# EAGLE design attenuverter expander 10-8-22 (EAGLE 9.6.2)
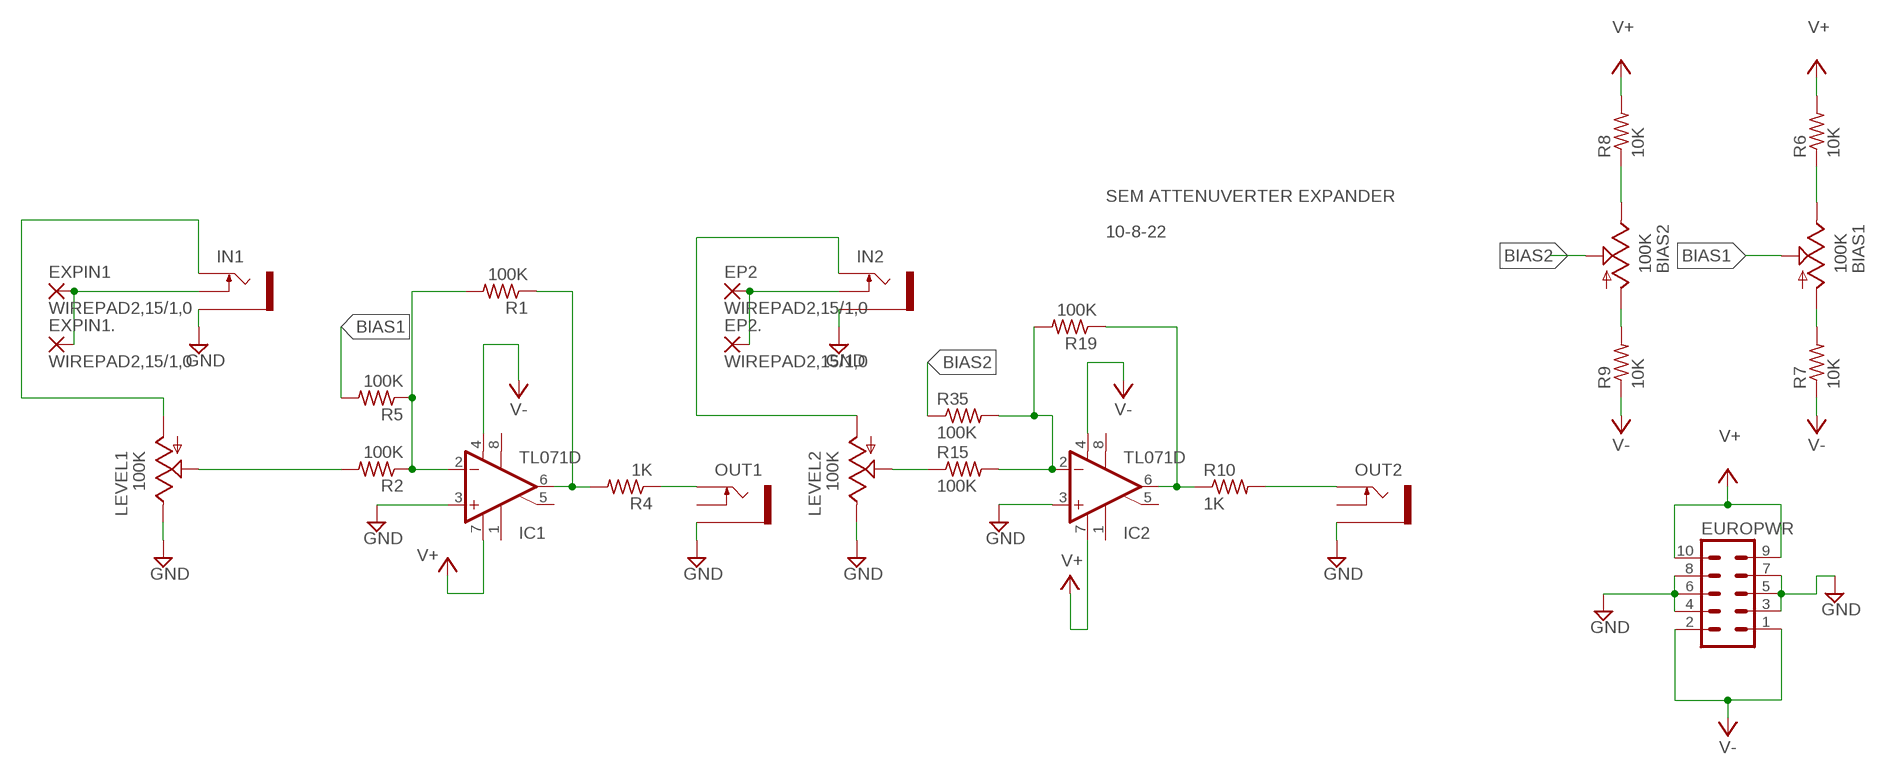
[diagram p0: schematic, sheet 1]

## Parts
BIAS1  100K  9MM_SNAP-IN_POT_  [9MM_SNAP-IN_POT]
BIAS2  100K  9MM_SNAP-IN_POT_  [9MM_SNAP-IN_POT]
EP2  WIREPAD2,15/1,0  [2,15/1,0]
EP2.  WIREPAD2,15/1,0  [2,15/1,0]
EUROPWR  EURO_POWER_HEADERREGULAR  [EURO_POWER_HEADER]
EXPIN1  WIREPAD2,15/1,0  [2,15/1,0]
EXPIN1.  WIREPAD2,15/1,0  [2,15/1,0]
IC1  TL071D  [SO08]
IC2  TL071D  [SO08]
IN1  THONKICONNNEW  [WQP-PJ301M-12_JACK]
IN2  THONKICONNNEW  [WQP-PJ301M-12_JACK]
LEVEL1  100K  9MM_SNAP-IN_POT_  [9MM_SNAP-IN_POT]
LEVEL2  100K  9MM_SNAP-IN_POT_  [9MM_SNAP-IN_POT]
OUT1  THONKICONNNEW  [WQP-PJ301M-12_JACK]
OUT2  THONKICONNNEW  [WQP-PJ301M-12_JACK]
R1  100K  R-US_0204/7  [0204/7]
R2  100K  R-US_0204/7  [0204/7]
R4  1K  R-US_0204/7  [0204/7]
R5  100K  R-US_0204/7  [0204/7]
R6  10K  R-US_0204/7  [0204/7]
R7  10K  R-US_0204/7  [0204/7]
R8  10K  R-US_0204/7  [0204/7]
R9  10K  R-US_0204/7  [0204/7]
R10  1K  R-US_0204/2V  [0204V]
R15  100K  R-US_0204/7  [0204/7]
R19  100K  R-US_0204/7  [0204/7]
R35  100K  R-US_0204/2V  [0204V]

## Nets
BIAS1: BIAS1.2(S) R5.2
BIAS2: BIAS2.2(S) R35.1
GND: EUROPWR.3 EUROPWR.4 EUROPWR.5 EUROPWR.6 EUROPWR.7 EUROPWR.8 IC1.3(+IN) IC2.3(+IN) IN1.P$3_SLEEVE(SLEEVE) IN2.P$3_SLEEVE(SLEEVE) LEVEL1.3(E) LEVEL2.3(E) OUT1.P$3_SLEEVE(SLEEVE) OUT2.P$3_SLEEVE(SLEEVE)
N$1: BIAS2.3(E) R8.1
N$2: BIAS2.1(A) R9.2
N$3: BIAS1.1(A) R7.2
N$4: BIAS1.3(E) R6.1
N$5: IC1.2(-IN) R1.2 R2.1 R5.1
N$6: IC1.6(OUT) R1.1 R4.2
N$7: IC2.2(-IN) R15.2 R19.2 R35.2
N$8: LEVEL1.2(S) R2.2
N$9: IC2.6(OUT) R10.1 R19.1
N$10: LEVEL2.2(S) R15.1
N$11: EXPIN1.1(P) EXPIN1..1(P) IN1.P$2_SWITCH(SWITCH)
N$12: EP2.1(P) EP2..1(P) IN2.P$2_SWITCH(SWITCH)
N$13: IN2.P$1_TIP(TIP) LEVEL2.1(A)
N$14: IN1.P$1_TIP(TIP) LEVEL1.1(A)
N$15: OUT2.P$1_TIP(TIP) R10.2
N$16: OUT1.P$1_TIP(TIP) R4.1
V+: EUROPWR.9 EUROPWR.10 IC1.7(V+) IC2.7(V+) R6.2 R8.2
V-: EUROPWR.1 EUROPWR.2 IC1.4(V-) IC2.4(V-) R7.1 R9.1
Unconnected: IC1.1(ON1) IC1.5(ON2) IC1.8(OPT) IC2.1(ON1) IC2.5(ON2) IC2.8(OPT) OUT1.P$2_SWITCH(SWITCH) OUT2.P$2_SWITCH(SWITCH)

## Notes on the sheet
- SEM ATTENUVERTER EXPANDER
- 10-8-22

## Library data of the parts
BIAS1 BIAS2 LEVEL1 LEVEL2 = MusicThingModular:9MM_SNAP-IN_POT: 9mm vertical snap-in pot, Alpha / Panasonic style
EP2 EP2. EXPIN1 EXPIN1. = wirepad:WIREPAD: Wire PAD connect wire on PCB
EUROPWR = MusicThingModular:EURO_POWER_HEADER: Power Header 10 pin power header for Eurorack Power Supplies Variants with fatter pads for easier soldering, and the LOCK variant which has 5mil offset pins to hold the component in place before soldering
IC1 IC2 = linear:TL071: OP AMP
IN1 IN2 OUT1 OUT2 = MusicThingModular-CL:THONKICONN: 3.5mm socket for Eurorack modular synths
R1 R2 R4 R5 = rcl:R-US_: RESISTOR, American symbol
R6-R10 R15 R19 R35 = adafruit:R-US_: RESISTOR, American symbol

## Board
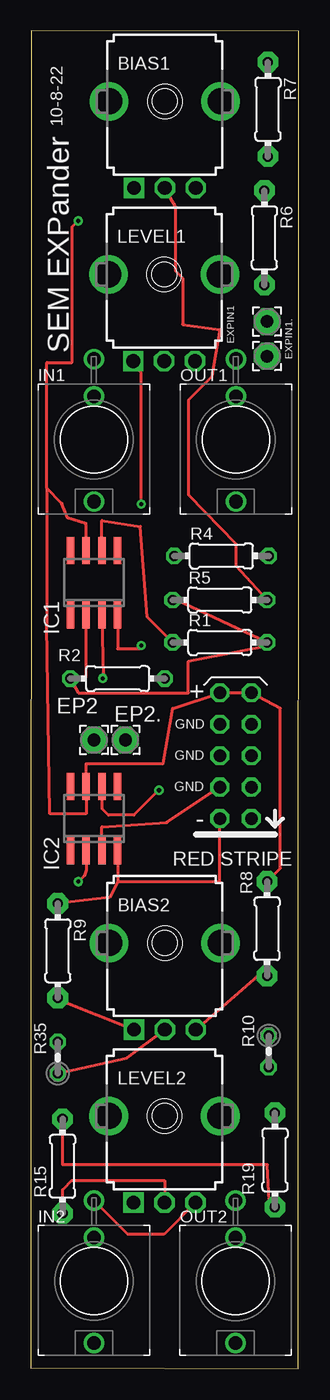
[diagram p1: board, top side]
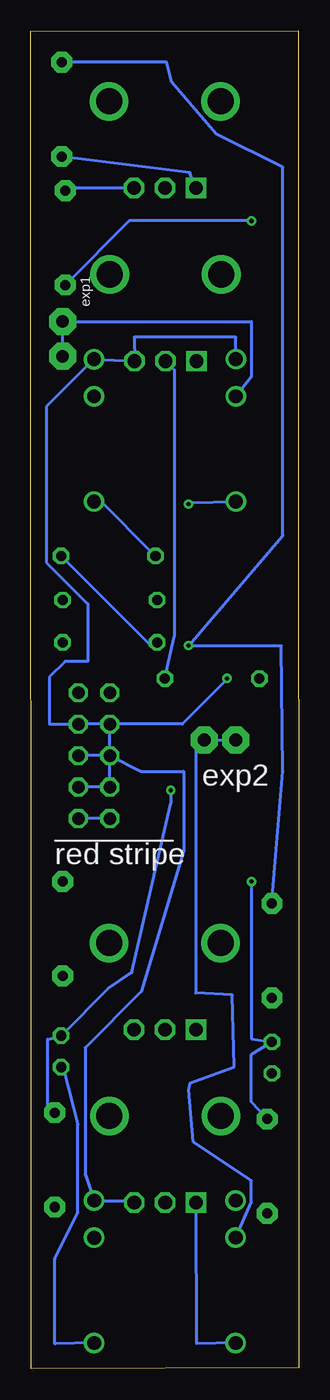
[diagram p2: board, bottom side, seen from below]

Size 21.61 x 108 mm. Coordinates in mm from the lower left corner, seen from the top.
Outline: 0,0.06 21.59,0 21.61,108 0.02,108 0,0.06
Copper layers (1*16): Top 0.035mm / dielectric 1.5mm / Bottom 0.035mm
Design rules "default": minimum track width 6mil, minimum drill 0.35mm, track to track 6mil, track to pad 6mil, pad to pad 6mil, via to via 6mil, smd to smd 6mil, copper to edge 40mil, drill to drill 6mil, minimum pad ring 10mil, minimum via ring 8mil, stop-mask expansion 4mil, vias tented up to drill 0mil, thermal gap 10mil

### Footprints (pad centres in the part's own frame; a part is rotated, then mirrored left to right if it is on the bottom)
9MM_SNAP-IN_POT = drill 1.1 square: 1 -2.5,-7 | drill 1.1 octagon: 2 0,-7; 3 2.5,-7 | drill 2.1 pad 2.794: CHASSIS1 -4.5,0; CHASSIS2 4.5,0
2,15/1,0 = drill 1.016 pad 2.159 octagon: 1 0,0
EURO_POWER_HEADER = drill 1.016 octagon: 1 -5.08,-1.27; 2 -5.08,1.27; 3 -2.54,-1.27; 4 -2.54,1.27; 5 0,-1.27; 6 0,1.27; 7 2.54,-1.27; 8 2.54,1.27; 9 5.08,-1.27; 10 5.08,1.27
SO08 = smd 0.6 x 2.2: 1 -1.905,-2.6; 2 -0.635,-2.6; 3 0.635,-2.6; 4 1.905,-2.6; 5 1.905,2.6; 6 0.635,2.6; 7 -0.635,2.6; 8 -1.905,2.6
WQP-PJ301M-12_JACK = drill 1.1: P$1_TIP 0,5; P$2_SWITCH 0,-3.5; P$3_SLEEVE 0,-6.5
0204/7 = drill 0.813 octagon: 1 -3.81,0; 2 3.81,0
0204/7' = drill 0.813 pad 1.676 octagon: 1 -3.81,0; 2 3.81,0
0204V = drill 0.813 octagon: 1 -1.27,0; 2 1.27,0

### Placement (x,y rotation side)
BIAS1  10.8,102.32 0 top
BIAS2  10.8,34.36 0 top
EP2  5.09,50.76 0 top
EP2.  7.63,50.76 0 top
EUROPWR  16.52,49.49 90 top
EXPIN1  19.06,81.74 0 top
EXPIN1.  19.06,84.54 0 top
IC1  5.09,63.46 0 top
IC2  5.09,44.41 0 top
IN1  5.08,75 180 top
IN2  5.09,7.07 180 top
LEVEL1  10.75,88.35 0 top
LEVEL2  10.78,20.39 0 top
OUT1  16.54,75 180 top
OUT2  16.51,7.06 180 top
R1  15.25,58.63 0 top
R2  6.99,55.71 0 top
R4  15.37,65.61 0 top
R5  15.25,62.06 0 top
R6  10K  [0204/7']  18.84,91.3 270 top
R7  10K  [0204/7']  19.13,101.68 270 top
R8  10K  [0204/7']  19.06,35.52 90 top
R9  10K  [0204/7']  2.17,33.74 270 top
R10  19.18,25.61 270 top
R15  100K  [0204/7']  2.55,16.34 90 top
R19  100K  [0204/7']  19.69,16.85 270 top
R35  2.17,25.1 90 top

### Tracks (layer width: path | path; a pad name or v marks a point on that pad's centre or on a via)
BIAS1
  Top 0.254: R5.2 16.52,64.82 16.52,66.63 12.71,70.57 12.71,78.19 14.61,80.09 15.25,83.9 12.24,84.3 12.24,88.06 11.69,88.6 11.69,93.77 BIAS1.2
BIAS2
  Top 0.254: R35.1 7.77,25.1 BIAS2.2
GND  (via drill 0.35)
  Top 0.254: IC1.3 5.84,55.69 v5.79,55.72 | IC2.3 5.72,43.74 10.97,44.09 EUROPWR.4 | LEVEL2.3 10.74,10.85 7.81,10.85 IN2.P$3_SLEEVE
  Bottom 0.254: IN1.P$3_SLEEVE 5.08,83.27 13.29,83.27 13.25,81.36 | 13.25,81.36 LEVEL1.3 | v5.79,55.72 5.79,55.63 9.39,52.03 EUROPWR.8 | EUROPWR.8 EUROPWR.7 20.12,52.03 20.12,55.84 18.85,57.11 17.02,57.11 17.02,61.75 20.38,65.1 20.38,77.66 OUT1.P$3_SLEEVE 13.25,81.36 | EUROPWR.6 EUROPWR.8 | EUROPWR.6 EUROPWR.5 | EUROPWR.6 EUROPWR.4 EUROPWR.3 | LEVEL2.3 13.45,13.56 OUT2.P$3_SLEEVE 17.24,15.67 17.24,25.9 12.71,30.44 9.28,41.85 9.28,48.22 12.71,48.22 EUROPWR.6
N$1
  Top 0.254: R8.1 18.29,31.71 BIAS2.3
N$2
  Top 0.254: BIAS2.1 2.4,29.7 R9.2
N$3
  Bottom 0.254: BIAS1.1 8.79,96.57 R7.2
N$4
  Bottom 0.254: R6.1 18.16,95.32 BIAS1.3
N$5
  Top 0.254: IC1.2 4.45,55.84 R2.1 3.82,54.57 12.71,54.57 12.71,57.11 18.7,58.28 R1.2 11.73,62.06 R5.1
N$6
  Top 0.254: IC1.6 5.72,68.49 8.82,68 9.4,60.67 R1.1
  Bottom 0.254: R4.2 11.84,58.27 R1.1
N$7  (via drill 0.35)
  Top 0.254: IC2.2 4.46,40.24 4.29,39.8 v3.82,39.33 | R19.2 19.24,13.49 19.07,16.47 2.55,16.47 R15.2
  Bottom 0.254: R15.2 3.82,21.55 3.82,25.36 R35.2 3.82,26.63 v3.82,39.33
N$8
  Bottom 0.254: R2.2 10.03,59.12 10.03,80.62 LEVEL1.2
N$9  (via drill 0.35)
  Top 0.254: IC2.6 5.72,45.22 6.26,44.68 8.3,44.68 v10.33,46.7
  Bottom 0.254: R19.1 20.27,21.23 20.27,26.59 R10.1 15.38,30.68 13.48,31.98 10.33,45.63 v10.33,46.7
N$10
  Top 0.254: R15.1 2.55,14.43 3.31,15.2 10.78,15.2 LEVEL2.2
N$11
  Bottom 0.254: IN1.P$2_SWITCH 3.82,80.08 3.82,84.54 EXPIN1..1 EXPIN1.1
N$12
  Bottom 0.254: EP2.1 EP2..1 8.32,50.06 8.32,30.33 5.35,30.17 5.22,24.36 8.75,23.06 8.89,22.52 8.5,18.31 3.82,15.2 3.82,13.42 IN2.P$2_SWITCH
N$13
  Bottom 0.254: IN2.P$1_TIP 8.24,2 LEVEL2.1
N$14  (via drill 0.35)
  Top 0.254: v8.9,69.81 8.9,80.36 LEVEL1.1
  Bottom 0.254: IN1.P$1_TIP 8.78,69.93 v8.9,69.81
N$15
  Bottom 0.254: OUT2.P$1_TIP 19.69,1.99 19.69,8.85 17.82,12.59 17.82,19.71 18.98,24.14 R10.2
N$16
  Bottom 0.254: OUT1.P$1_TIP 16.2,70.25 R4.1
V+  (via drill 0.35)
  Top 0.254: 1.28,71.08 2.5,69.85 2.97,68.69 4.44,68.25 4.45,68.03 IC1.7 | 1.28,71.08 1.28,81.24 3.31,81.24 3.31,92.16 v3.82,92.67 | 1.28,71.08 1.28,60.03 1.53,44.79 4.45,44.79 IC2.7 4.45,48.85 10.67,48.85 11.44,53.3 EUROPWR.10 EUROPWR.9 20.12,53.3 20.12,40.39 R8.2
  Bottom 0.254: v3.82,92.67 13.67,92.67 R6.2
V-  (via drill 0.35)
  Top 0.254: IC1.4 6.99,58.12 8.9,58.12 v8.9,58.38 | IC2.4 6.99,39.33 | 6.99,39.33 6.36,38.06 R9.1 | 6.99,39.33 15.25,39.33 EUROPWR.2
  Bottom 0.254: R7.1 10.69,105.49 10.29,103.91 6.66,99.68 1.28,96.98 1.28,67.27 v8.9,58.38 1.39,58.38 1.28,48.22 R9.1 | EUROPWR.2 EUROPWR.1

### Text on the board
tNames: 10-8-22 | SEM EXPander
bNames: exp1 | exp2 | red stripe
